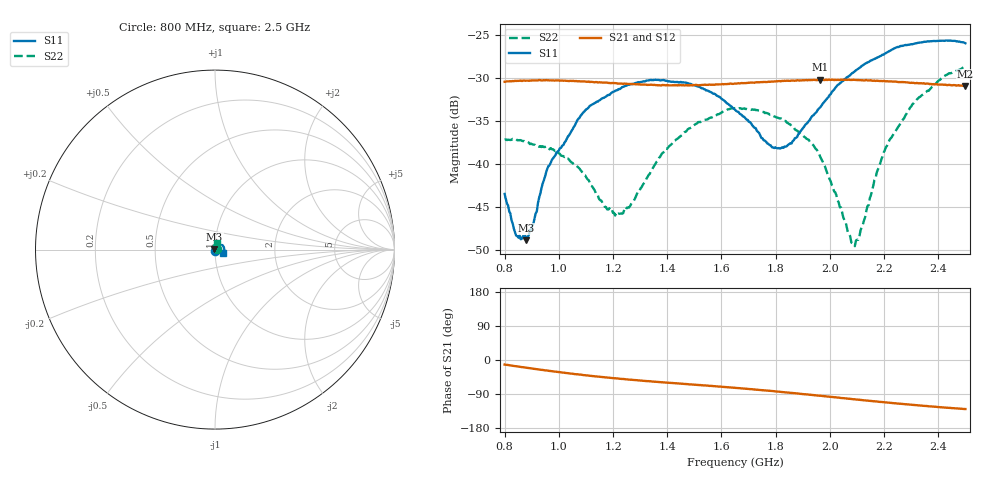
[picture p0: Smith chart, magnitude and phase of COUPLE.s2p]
!Agilent Technologies,N5234A,MY52241180,A.10.00.00
!Agilent N5234A: A.10.00.00
!Date: Tuesday, August 18, 2015 23:53:23
!Correction: S11(Full 2 Port(1,2))
!S21(Full 2 Port(1,2))
!S12(Full 2 Port(1,2))
!S22(Full 2 Port(1,2))
!S2P File: Measurements: S11, S21, S12, S22:
# Hz S  dB  R 50
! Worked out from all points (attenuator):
!   401 points, 800 MHz to 2.5 GHz, reference 50 ohm
!   highest |S21| = -30.17 dB at 1.964 GHz (marker M1); lowest = -30.9 dB at 2.5 GHz (marker M2)
!   lowest |S11| = -48.9 dB at 880.8 MHz (marker M3), VSWR 1.01, Z = 49.7 + j0.114 ohm
!   |S11| at or under -10 dB: start of sweep to end of sweep
!   |S22| runs from -49.6 to -28.6 dB; largest |S21 - S12| = 0.00031
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8e8  -43.48 -105.7  -30.42 -11.9  -30.42 -12.0  -37.17 11.7
8.425e8  -48.33 -147.1  -30.33 -16.5  -30.34 -16.5  -37.11 8.6
8.8075e8  -48.88 161.4  -30.29 -20.5  -30.29 -20.5  -37.46 4.8
9.0625e8  -46.94 128.5  -30.26 -23.2  -30.28 -23.0  -37.74 1.2
9.615e8  -40.25 95.6  -30.25 -28.4  -30.29 -28.4  -38.10 -5.7
1.08475e9  -34.23 58.1  -30.39 -39.0  -30.39 -39.2  -40.89 -9.4
1.174e9  -32.15 40.1  -30.52 -46.0  -30.55 -46.0  -45.01 8.7
1.225e9  -31.28 28.4  -30.63 -49.4  -30.64 -49.5  -45.80 36.7
1.2675e9  -30.69 19.5  -30.69 -52.1  -30.71 -52.3  -44.62 56.2
1.3695e9  -30.22 -2.4  -30.82 -58.2  -30.81 -58.1  -39.30 65.3
1.5055e9  -30.90 -35.0  -30.78 -65.2  -30.83 -65.4  -35.34 56.7
1.65e9  -33.67 -77.5  -30.62 -73.5  -30.64 -73.4  -33.49 37.7
1.8115e9  -38.14 -162.6  -30.34 -83.5  -30.38 -83.7  -34.67 15.3
1.85825e9  -37.62 164.7  -30.28 -86.9  -30.34 -86.8  -35.57 8.6
1.93475e9  -34.43 123.7  -30.23 -92.2  -30.24 -92.3  -37.68 -1.2
1.9645e9  -33.39 111.0  -30.17 -94.2  -30.21 -94.5  -39.17 -1.6
2.08775e9  -29.31 72.4  -30.19 -103.5  -30.22 -103.6  -49.29 53.9
2.11325e9  -28.72 65.7  -30.24 -105.5  -30.27 -105.4  -47.71 91.0
2.17275e9  -27.65 50.9  -30.30 -109.3  -30.34 -109.6  -41.00 106.2
2.2195e9  -26.85 39.3  -30.39 -112.7  -30.39 -112.8  -37.23 107.7
2.3215e9  -25.92 16.8  -30.56 -119.5  -30.58 -119.4  -32.47 96.0
2.5e9  -25.94 -22.2  -30.91 -129.4  -30.90 -129.4  -28.64 68.4
